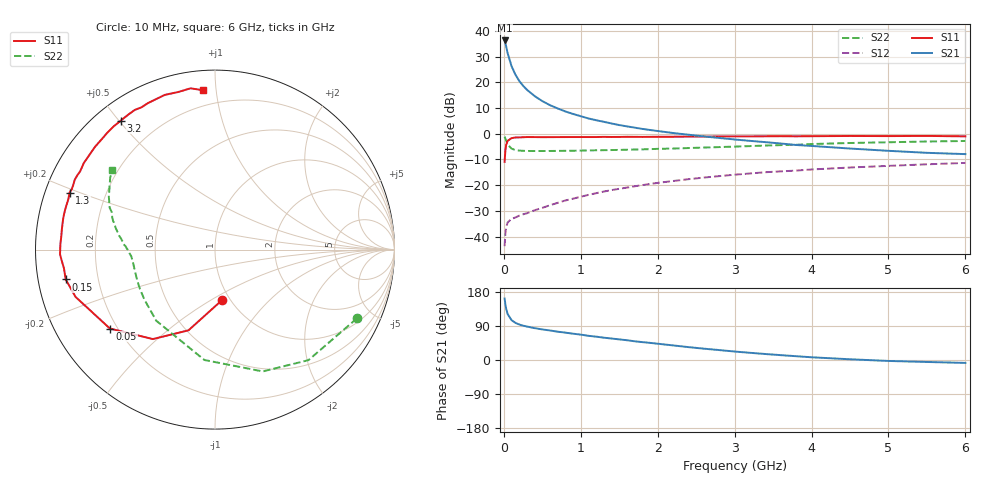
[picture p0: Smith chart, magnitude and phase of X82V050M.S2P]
! SIEMENS Small Signal Semiconductors
! BFP136W
! Si NPN RF Bipolar Junction Transistor in SOT343
! VCE = 2 V  IC = 50 mA
! Common Emitter S-Parameters:  September  1994
# GHz  S  MA  R  50
!  f  S11  S21  S12  S22
! GHz  MAG  ANG  MAG  ANG  MAG  ANG  MAG  ANG
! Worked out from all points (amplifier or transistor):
!   40 points, 10 MHz to 6 GHz, reference 50 ohm
!   highest |S21| = 36.3 dB at 10 MHz (marker M1)
!   |S21| within 3 dB of that: start of sweep to 34.9 MHz
!   unconditionally stable (mu >= 1): 579.6 MHz to 2.835 GHz
!   at 200 MHz: K = 0.56, MSG = 26.2 dB, |S12| = -31.9 dB
!   at 1.5 GHz: K = 1.12, MAG = 10.3 dB, |S12| = -21.4 dB
!   at 6 GHz: K = 0.98, MSG = 1.7 dB, |S12| = -11.3 dB
!   S11 on the Smith chart (normalised r, x): 10 MHz: 0.92, -0.56; 50 MHz: 0.17, -0.32; 150 MHz: 0.08, -0.10; 1.3 GHz: 0.07, +0.19; 3.2 GHz: 0.07, +0.51; 6 GHz: 0.11, +0.92
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0.01  0.2846 -82.2  65.45 162.3  0.0065 71.5  0.8784 -25.9
0.02  0.4736 -108.2  57.73 147.1  0.0115 60.3  0.8065 -49.8
0.03  0.607 -124.8  49.97 135.7  0.0152 50.6  0.7292 -68.6
0.05  0.7323 -143.1  36.73 121.0  0.0189 39.4  0.6178 -95.5
0.1  0.8207 -161.3  20.73 105.2  0.0221 31.9  0.5139 -129.6
0.15  0.8481 -168.7  14.18 98.1  0.0235 31.7  0.4819 -144.8
0.2  0.8481 -173.0  10.66 93.7  0.0255 34.0  0.4712 -153.1
0.25  0.8572 -176.2  8.605 90.6  0.0271 36.8  0.4663 -158.4
0.3  0.8639 -178.3  7.198 88.3  0.0284 39.5  0.4629 -162.0
0.4  0.8619 177.8  5.42 84.1  0.0325 44.2  0.4616 -166.7
0.5  0.8595 175.0  4.323 80.7  0.0362 48.2  0.4618 -169.7
0.6  0.8606 172.8  3.603 77.9  0.0407 50.9  0.4628 -171.6
0.7  0.8617 170.3  3.109 74.7  0.0453 53.7  0.4644 -172.9
0.9  0.8639 166.7  2.431 69.4  0.0546 56.1  0.468 -175.4
1.1  0.8636 162.3  1.988 63.8  0.0647 57.6  0.474 -176.9
1.3  0.8702 158.6  1.712 58.9  0.0752 58.3  0.4799 -178.4
1.7  0.8717 151.6  1.317 49.4  0.0951 57.5  0.4939 178.8
2.2  0.8762 143.2  1.035 38.5  0.1205 54.7  0.5162 175.1
3.2  0.8899 126.2  0.728 19.0  0.1688 46.2  0.5757 166.1
4.5  0.9062 108.0  0.516 1.9  0.2205 34.1  0.6616 153.4
5.5  0.9088 98.6  0.426 -5.2  0.2547 26.0  0.7073 145.7
6  0.8906 94.4  0.402 -7.7  0.2711 21.5  0.724 142.4
